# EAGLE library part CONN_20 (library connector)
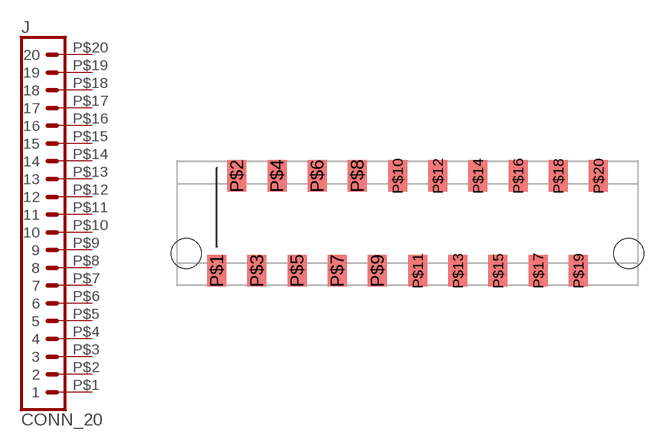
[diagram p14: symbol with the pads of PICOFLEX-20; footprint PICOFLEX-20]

Designator prefix J

## CONN_20PICOFLEX  [PICOFLEX-20]
P$1  1  pas
P$2  2  pas
P$3  3  pas
P$4  4  pas
P$5  5  pas
P$6  6  pas
P$7  7  pas
P$8  8  pas
P$9  9  pas
P$10  10  pas
P$11  11  pas
P$12  12  pas
P$13  13  pas
P$14  14  pas
P$15  15  pas
P$16  16  pas
P$17  17  pas
P$18  18  pas
P$19  19  pas
P$20  20  pas

## Footprint PICOFLEX-20 (pad centres in mm)
smd 1.2 x 2: P$1 0,0; P$2 1.27,6; P$3 2.54,0; P$4 3.81,6; P$5 5.08,0; P$6 6.35,6; P$7 7.62,0; P$8 8.89,6; P$9 10.16,0; P$10 11.43,6; P$11 12.7,0; P$12 13.97,6; P$13 15.24,0; P$14 16.51,6; P$15 17.78,0; P$16 19.05,6; P$17 20.32,0; P$18 21.59,6; P$19 22.86,0; P$20 24.13,6
hole 1.9 at -1.93,1.1
hole 1.9 at 26.05,1.1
